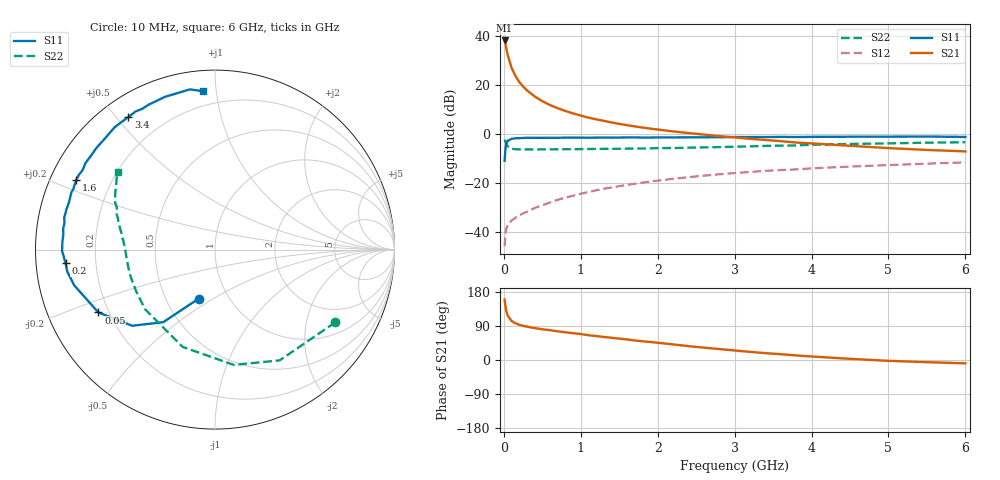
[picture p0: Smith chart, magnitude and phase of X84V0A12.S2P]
! SIEMENS Small Signal Semiconductors
! BFP136W
! Si NPN RF Bipolar Junction Transistor in SOT343
! VCE = 4 V  IC = 120 mA
! Common Emitter S-Parameters:  September  1994
# GHz  S  MA  R  50
!  f  S11  S21  S12  S22
! GHz  MAG  ANG  MAG  ANG  MAG  ANG  MAG  ANG
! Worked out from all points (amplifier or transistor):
!   40 points, 10 MHz to 6 GHz, reference 50 ohm
!   highest |S21| = 38.4 dB at 10 MHz (marker M1)
!   |S21| within 3 dB of that: start of sweep to 30.38 MHz
!   unconditionally stable (mu >= 1): 500.7 MHz to 2.932 GHz
!   at 200 MHz: K = 0.71, MSG = 27.2 dB, |S12| = -33.1 dB
!   at 1.5 GHz: K = 1.10, MAG = 10.8 dB, |S12| = -21.2 dB
!   at 6 GHz: K = 0.97, MSG = 2.2 dB, |S12| = -11.4 dB
!   S11 on the Smith chart (normalised r, x): 10 MHz: 0.72, -0.43; 50 MHz: 0.16, -0.25; 200 MHz: 0.09, -0.05; 1.6 GHz: 0.08, +0.24; 3.4 GHz: 0.08, +0.54; 6 GHz: 0.11, +0.92
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0.01  0.2888 -108.5  82.94 159.7  0.0052 67.9  0.7829 -31.2
0.02  0.4964 -125.5  70.59 142.9  0.0089 57.0  0.7146 -59.7
0.03  0.6271 -137.4  59.1 131.1  0.0115 50.0  0.6511 -80.7
0.05  0.7383 -151.7  41.88 117.2  0.0141 40.2  0.5712 -108.4
0.1  0.8095 -165.8  23.03 103.1  0.0173 37.5  0.5121 -139.5
0.15  0.832 -171.5  15.65 96.9  0.0198 41.0  0.4969 -152.1
0.2  0.8363 -174.8  11.76 93.1  0.0222 43.3  0.4935 -159.0
0.25  0.8443 -177.6  9.493 90.2  0.0243 45.5  0.4936 -163.4
0.3  0.8521 -179.4  7.932 88.1  0.0264 48.1  0.4925 -166.4
0.4  0.8514 177.0  5.974 84.3  0.0313 52.0  0.4933 -170.4
0.5  0.8491 174.4  4.763 81.1  0.0357 54.8  0.4941 -173.1
0.6  0.8538 172.2  3.977 78.6  0.0405 56.7  0.4952 -175.0
0.7  0.8518 169.9  3.426 75.6  0.0461 58.5  0.4965 -176.3
0.9  0.8573 166.2  2.685 70.7  0.0558 60.1  0.4988 -178.9
1.1  0.855 162.0  2.197 65.4  0.0665 60.5  0.5024 179.4
1.6  0.8648 153.2  1.543 54.3  0.0926 59.1  0.5114 175.4
2.2  0.8666 143.0  1.151 41.1  0.1236 54.9  0.5264 170.8
3.2  0.8811 126.1  0.812 21.5  0.1705 45.6  0.5685 162.1
3.4  0.8825 123.2  0.77 18.1  0.18 43.4  0.5815 160.3
4.5  0.8957 108.1  0.584 3.1  0.2197 33.3  0.6374 150.8
5.5  0.9037 98.9  0.481 -5.7  0.2522 25.6  0.6764 144.2
6  0.8853 94.5  0.449 -8.8  0.2682 21.3  0.6912 141.4
